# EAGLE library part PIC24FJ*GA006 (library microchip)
64/80/100-Pin General Purpose, 16-Bit Flash Microcontrollers Source: http://ww1.microchip.com/downloads/en/DeviceDoc/39747d.pdf
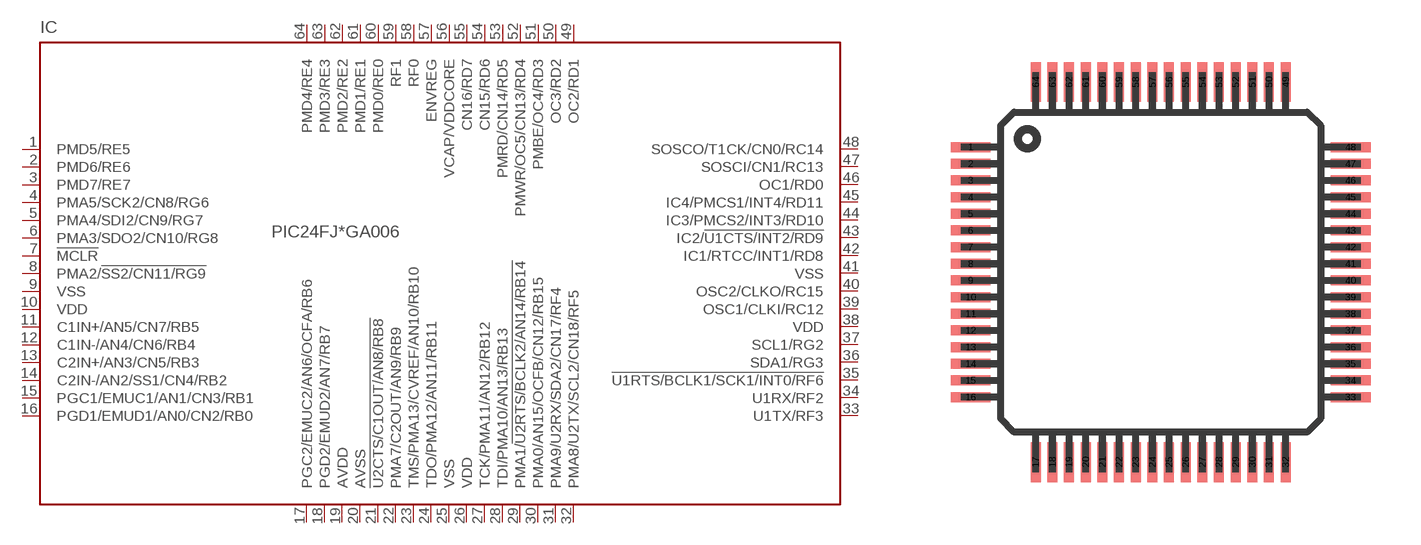
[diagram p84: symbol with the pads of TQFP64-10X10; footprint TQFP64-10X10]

Designator prefix IC

## PIC24FJ128GA006 (MF: MICROCHIP; MPN: PIC24FJ128GA006-I/PT; OC_FARNELL: 1146519; OC_NEWARK: 56K7337), PIC24FJ64GA006 (MPN: PIC24FJ64GA006-I/PT; OC_FARNELL: 1146524; OC_NEWARK: 56K7343), PIC24FJ69GA006 (OC_FARNELL: unknown; OC_NEWARK: unknown)  [TQFP64-10X10]
1  PMD5/RE5
2  PMD6/RE6
3  PMD7/RE7
4  PMA5/SCK2/CN8/RG6
5  PMA4/SDI2/CN9/RG7
6  PMA3/SDO2/CN10/RG8
7  !MCLR
8  PMA2/!SS2/CN11/RG9
9  VSS  pwr
10  VDD  pwr
11  C1IN+/AN5/CN7/RB5
12  C1IN-/AN4/CN6/RB4
13  C2IN+/AN3/CN5/RB3
14  C2IN-/AN2/SS1/CN4/RB2
15  PGC1/EMUC1/AN1/CN3/RB1
16  PGD1/EMUD1/AN0/CN2/RB0
17  PGC2/EMUC2/AN6/OCFA/RB6
18  PGD2/EMUD2/AN7/RB7
19  AVDD  pwr
20  AVSS  pwr
21  !U2CTS/C1OUT/AN8/RB8
22  PMA7/C2OUT/AN9/RB9
23  TMS/PMA13/CVREF/AN10/RB10
24  TDO/PMA12/AN11/RB11
25  VSS  pwr
26  VDD  pwr
27  TCK/PMA11/AN12/RB12
28  TDI/PMA10/AN13/RB13
29  PMA1/!U2RTS/BCLK2/AN14/RB14
30  PMA0/AN15/OCFB/CN12/RB15
31  PMA9/U2RX/SDA2/CN17/RF4
32  PMA8/U2TX/SCL2/CN18/RF5
33  U1TX/RF3
34  U1RX/RF2
35  !U1RTS/BCLK1/SCK1/INT0/RF6
36  SDA1/RG3
37  SCL1/RG2
38  VDD  pwr
39  OSC1/CLKI/RC12
40  OSC2/CLKO/RC15
41  VSS  pwr
42  IC1/RTCC/INT1/RD8
43  IC2/!U1CTS/INT2/RD9
44  IC3/PMCS2/INT3/RD10
45  IC4/PMCS1/INT4/RD11
46  OC1/RD0
47  SOSCI/CN1/RC13
48  SOSCO/T1CK/CN0/RC14
49  OC2/RD1
50  OC3/RD2
51  PMBE/OC4/RD3
52  PMWR/OC5/CN13/RD4
53  PMRD/CN14/RD5
54  CN15/RD6
55  CN16/RD7
56  VCAP/VDDCORE
57  ENVREG
58  RF0
59  RF1
60  PMD0/RE0
61  PMD1/RE1
62  PMD2/RE2
63  PMD3/RE3
64  PMD4/RE4

## Footprint TQFP64-10X10 (pad centres in mm)
Thin Quad Flat Pack package type TQ
smd 1.2 x 0.3: 1 -5.7,3.75; 2 -5.7,3.25; 3 -5.7,2.75; 4 -5.7,2.25; 5 -5.7,1.75; 6 -5.7,1.25; 7 -5.7,0.75; 8 -5.7,0.25; 9 -5.7,-0.25; 10 -5.7,-0.75; 11 -5.7,-1.25; 12 -5.7,-1.75; 13 -5.7,-2.25; 14 -5.7,-2.75; 15 -5.7,-3.25; 16 -5.7,-3.75; 33 5.7,-3.75; 34 5.7,-3.25; 35 5.7,-2.75; 36 5.7,-2.25; 37 5.7,-1.75; 38 5.7,-1.25; 39 5.7,-0.75; 40 5.7,-0.25; 41 5.7,0.25; 42 5.7,0.75; 43 5.7,1.25; 44 5.7,1.75; 45 5.7,2.25; 46 5.7,2.75; 47 5.7,3.25; 48 5.7,3.75
smd 0.3 x 1.2: 17 -3.75,-5.7; 18 -3.25,-5.7; 19 -2.75,-5.7; 20 -2.25,-5.7; 21 -1.75,-5.7; 22 -1.25,-5.7; 23 -0.75,-5.7; 24 -0.25,-5.7; 25 0.25,-5.7; 26 0.75,-5.7; 27 1.25,-5.7; 28 1.75,-5.7; 29 2.25,-5.7; 30 2.75,-5.7; 31 3.25,-5.7; 32 3.75,-5.7; 49 3.75,5.7; 50 3.25,5.7; 51 2.75,5.7; 52 2.25,5.7; 53 1.75,5.7; 54 1.25,5.7; 55 0.75,5.7; 56 0.25,5.7; 57 -0.25,5.7; 58 -0.75,5.7; 59 -1.25,5.7; 60 -1.75,5.7; 61 -2.25,5.7; 62 -2.75,5.7; 63 -3.25,5.7; 64 -3.75,5.7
